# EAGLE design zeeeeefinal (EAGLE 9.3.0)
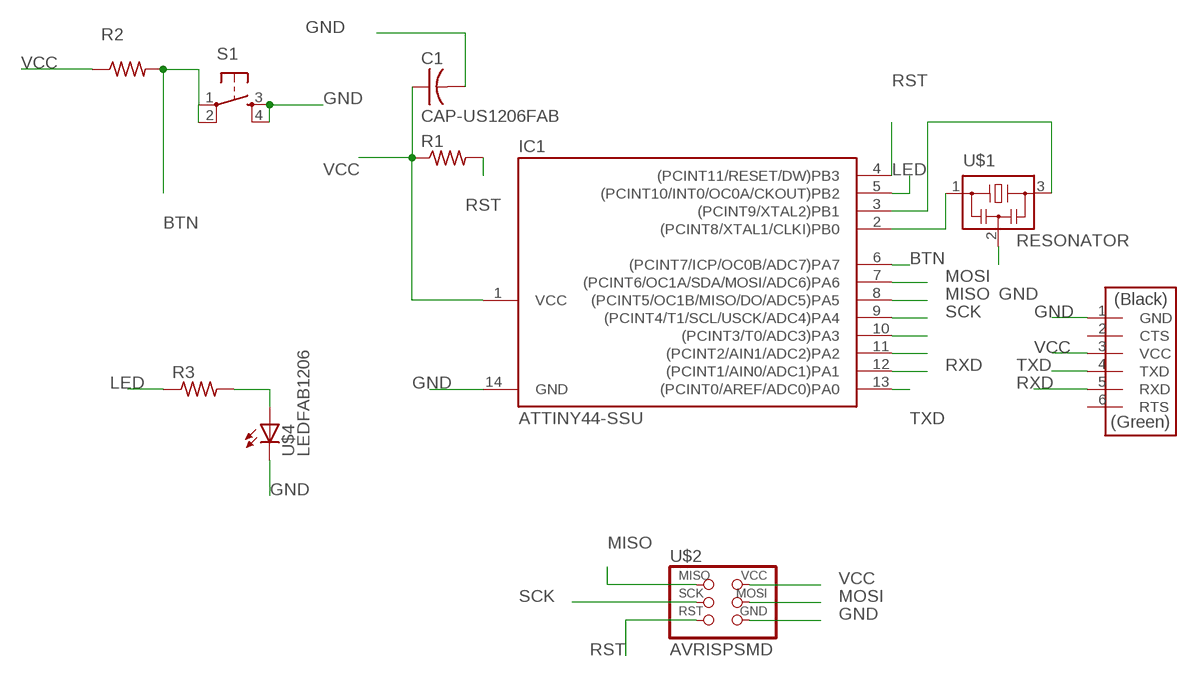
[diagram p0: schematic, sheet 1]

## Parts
C1  CAP-US1206FAB  [C1206FAB]
IC1  ATTINY44-SSU  [SOIC14]
R1  RES-US1206FAB  [R1206FAB]
R2  RES-US1206FAB  [R1206FAB]
R3  RES-US1206FAB  [R1206FAB]
S1  6MM_SWITCH6MM_SWITCH  [6MM_SWITCH]
U$1  RESONATOR  [EFOBM]
U$2  AVRISPSMD  [2X03SMD]
U$3  FTDI-SMD-HEADER  [1X06SMD]
U$4  LEDFAB1206  [LED1206FAB]

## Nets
BTN: IC1.6((PCINT7/ICP/OC0B/ADC7)PA7) R2.2 S1.1(P) S1.2(P1)
GND: C1.2 IC1.14(GND) S1.3(S) S1.4(S1) U$1.2 U$2.6(GND) U$3.1(GND) U$4.2(C)
LED: IC1.5((PCINT10/INT0/OC0A/CKOUT)PB2) R3.1
MISO: IC1.8((PCINT5/OC1B/MISO/DO/ADC5)PA5) U$2.1(MISO)
MOSI: IC1.7((PCINT6/OC1A/SDA/MOSI/ADC6)PA6) U$2.4(MOSI)
N$1: IC1.2((PCINT8/XTAL1/CLKI)PB0) U$1.1
N$2: IC1.3((PCINT9/XTAL2)PB1) U$1.3
N$3: R3.2 U$4.1(A)
N$7: IC1.10((PCINT3/T0/ADC3)PA3)
N$8: IC1.11((PCINT2/AIN1/ADC2)PA2)
RST: IC1.4((PCINT11/RESET/DW)PB3) R1.2 U$2.5(RST)
RXD: IC1.12((PCINT1/AIN0/ADC1)PA1) U$3.5(RXD)
SCK: IC1.9((PCINT4/T1/SCL/USCK/ADC4)PA4) U$2.3(SCK)
TXD: IC1.13((PCINT0/AREF/ADC0)PA0) U$3.4(TXD)
VCC: C1.1 IC1.1(VCC) R1.1 R2.1 U$2.2(VCC) U$3.3(VCC)
Unconnected: U$3.2(CTS) U$3.6(RTS)

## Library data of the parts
C1 = fab:CAP-US
IC1 = fab:ATTINY44
R1-R3 = fab:RES-US: Resistor (US Symbol)
S1 = fab:6MM_SWITCH: OMRON SWITCH
U$1 = fab:RESONATOR
U$2 = fab:AVRISP
U$3 = fab:FTDI-SMD-HEADER
U$4 = fab:LED: LED

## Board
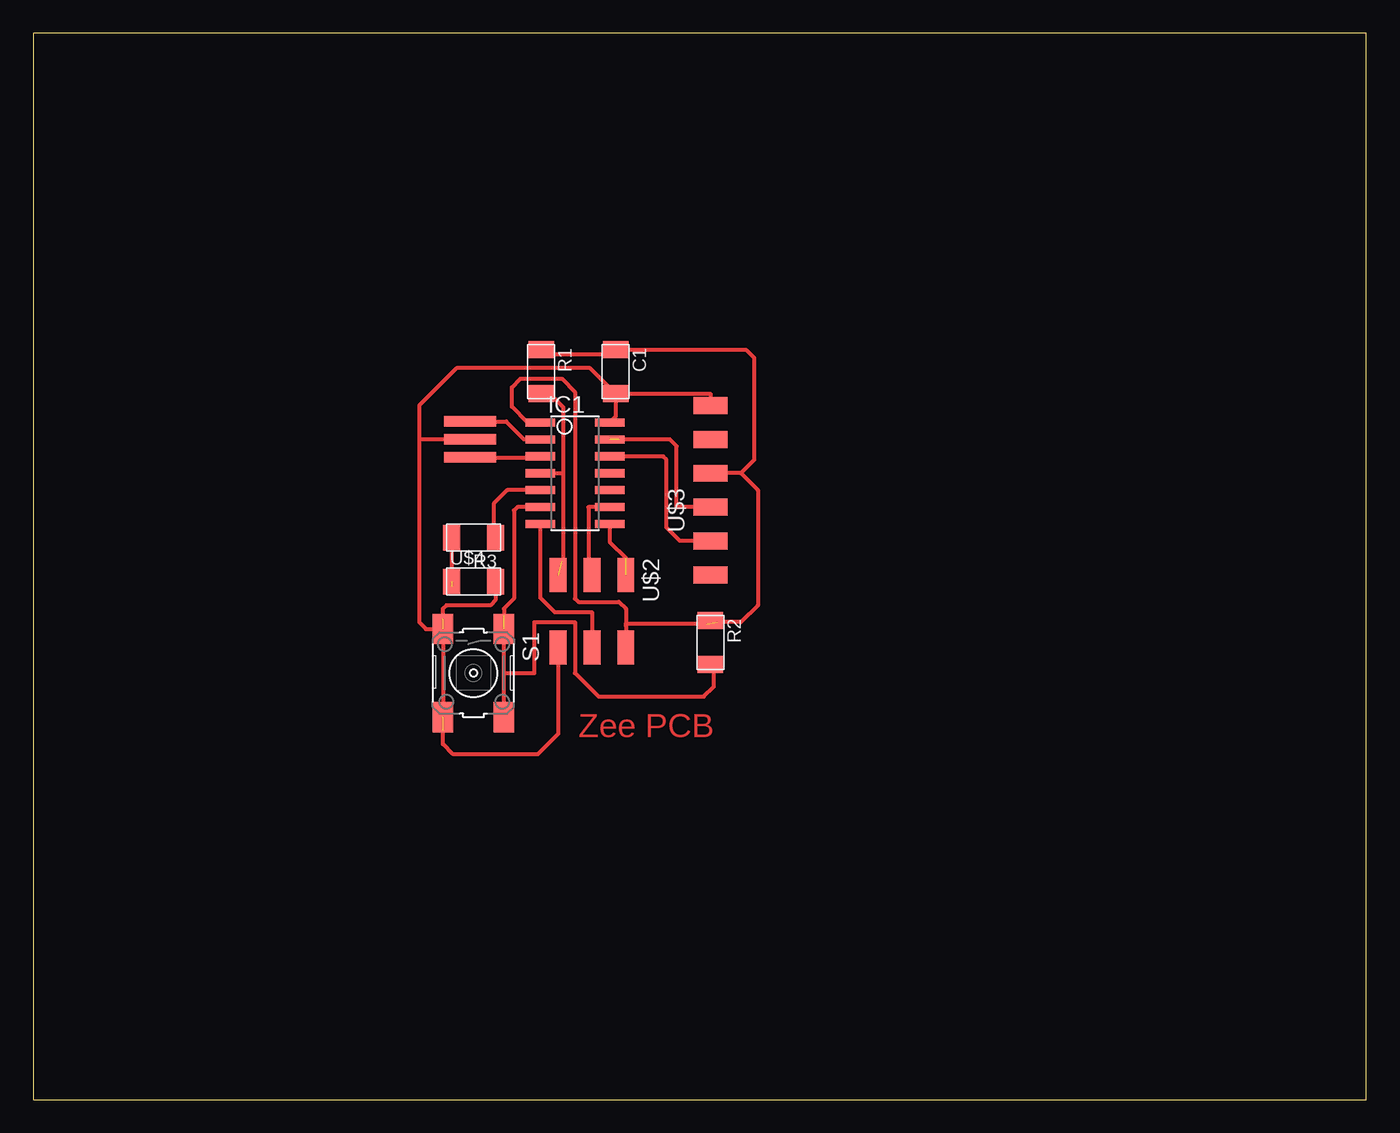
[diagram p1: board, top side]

Size 100 x 80 mm. Coordinates in mm from the lower left corner, seen from the top.
Outline: 0,0 100,0 100,80 0,80 0,0
Copper layers (1*16): Top 0.035mm / dielectric 1.5mm / Bottom 0.035mm
Design rules "default": minimum track width 6mil, minimum drill 0.35mm, track to track 6mil, track to pad 6mil, pad to pad 6mil, via to via 6mil, smd to smd 6mil, copper to edge 40mil, drill to drill 6mil, minimum pad ring 10mil, minimum via ring 8mil, stop-mask expansion 4mil, vias tented up to drill 0mil, thermal gap 10mil

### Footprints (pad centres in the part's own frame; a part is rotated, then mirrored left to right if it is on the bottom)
C1206FAB = smd 1.27 x 1.905: 1 -1.651,0; 2 1.651,0
SOIC14 = smd 0.61 x 2.21: 1 -3.81,-2.603; 2 -2.54,-2.603; 3 -1.27,-2.603; 4 0,-2.603; 5 1.27,-2.603; 6 2.54,-2.603; 7 3.81,-2.603; 8 3.81,2.603; 9 2.54,2.603; 10 1.27,2.603; 11 0,2.603; 12 -1.27,2.603; 13 -2.54,2.603; 14 -3.81,2.603
R1206FAB = smd 1.27 x 1.905: 1 -1.651,0; 2 1.651,0
6MM_SWITCH = smd 2.286 x 1.524: 1 -3.302,2.286; 2 3.302,2.286; 3 -3.302,-2.286; 4 3.302,-2.286
EFOBM = smd 0.8 x 3.9: 1 -1.35,0; 2 0,0; 3 1.35,0
2X03SMD = smd 2.54 x 1.27: 1 -2.54,2.54; 2 2.92,2.54; 3 -2.54,0; 4 2.92,0; 5 -2.54,-2.54; 6 2.92,-2.54
1X06SMD = smd 2.54 x 1.27: 1 0,6.35; 2 0,3.81; 3 0,1.27; 4 0,-1.27; 5 0,-3.81; 6 0,-6.35
LED1206FAB = smd 1.27 x 1.905: 1 -1.651,0; 2 1.651,0

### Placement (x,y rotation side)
C1  43.69,54.61 270 top
IC1  40.64,46.99 270 top
R1  38.1,54.61 270 top
R2  50.8,34.29 270 top
R3  33.02,42.16 180 top
S1  33.02,32 270 top
U$1  32.77,49.53 270 top
U$2  41.91,36.83 270 top
U$3  50.8,45.72 0 top
U$4  33.02,38.86 0 top

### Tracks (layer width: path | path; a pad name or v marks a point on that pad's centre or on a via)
BTN  (1 unrouted)
  Top 0.152: 51.05,32.38 R2.2
  Top 0.305: IC1.6 36.32,44.45 36.07,44.2 36.07,37.59 35.31,36.83 35.31,36.32 | S1.2 35.31,32 | 35.31,32 S1.1 | 35.31,32 37.59,32 37.59,35.81 40.64,35.81 40.64,32 42.42,30.23 50.29,30.23 51.05,30.99 51.05,32.38
GND  (2 unrouted)
  Top 0.305: U$1.2 28.96,49.53 | U$2.6 39.37,27.43 37.85,25.91 31.5,25.91 30.73,26.67 30.73,27.69 | U$4.2 34.67,37.47 34.29,37.08 30.99,37.08 30.73,36.83 30.73,36.07 | S1.4 S1.3 29.46,35.31 28.96,35.81 28.96,49.53 | C1.2 43.69,51.24 IC1.14 | C1.2 50.8,52.96 U$3.1 | C1.2 41.78,54.86 31.75,54.86 28.96,52.07 28.96,49.53
LED
  Top 0.305: IC1.5 35.56,45.72 34.54,44.7 34.54,42.29 R3.1
MISO  (1 unrouted)
  Top 0.305: IC1.8 43.24,41.85 44.45,40.64
MOSI
  Top 0.305: IC1.7 38.04,37.66 39.12,36.58 41.91,36.58 U$2.4
N$1
  Top 0.152: 36.83,49.53 IC1.2
  Top 0.305: U$1.1 35.48,50.88 36.83,49.53
N$2
  Top 0.152: 37.96,48.18 IC1.3
  Top 0.305: U$1.3 37.96,48.18
N$3  (1 unrouted)
  Top 0.152: 31.37,38.48 31.5,38.35
  Top 0.305: R3.2 31.37,38.48
RST  (1 unrouted)
  Top 0.152: 39.75,40.51 39.62,40.39 | R1.2 38.73,52.96
  Top 0.305: 39.75,46.99 39.75,46.23 39.75,40.51 | IC1.4 39.75,46.99 | 39.75,46.99 39.75,51.94 38.73,52.96
RXD
  Top 0.305: U$3.5 48.51,41.91 47.5,42.93 47.5,48.01 47.24,48.26 IC1.12
SCK
  Top 0.152: 41.4,39.62 41.4,39.88 41.66,39.62 U$2.3
  Top 0.305: IC1.9 41.66,44.45 41.66,39.62
TXD  (1 unrouted)
  Top 0.305: U$3.4 48.26,44.45 48.26,49.02 47.75,49.53 43.94,49.53
VCC  (1 unrouted)
  Top 0.152: C1.1 43.31,55.88 | 38.48,55.88 R1.1 | IC1.1 37.08,50.8
  Top 0.305: 53.09,46.99 U$3.3 | 53.09,46.99 54.36,45.72 54.36,37.08 53.09,35.81 51.31,35.81 | 53.09,46.99 54.1,48.01 54.1,55.63 53.47,56.26 C1.1 | R2.1 50.55,35.69 44.45,35.69 44.45,36.83 43.94,37.34 40.89,37.34 40.64,37.59 40.64,53.09 39.66,54.08 36.55,54.08 35.9,53.44 35.9,51.98 37.08,50.8 | 44.45,35.56 U$2.2 | 43.31,55.88 38.48,55.88

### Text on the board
Top: Zee PCB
